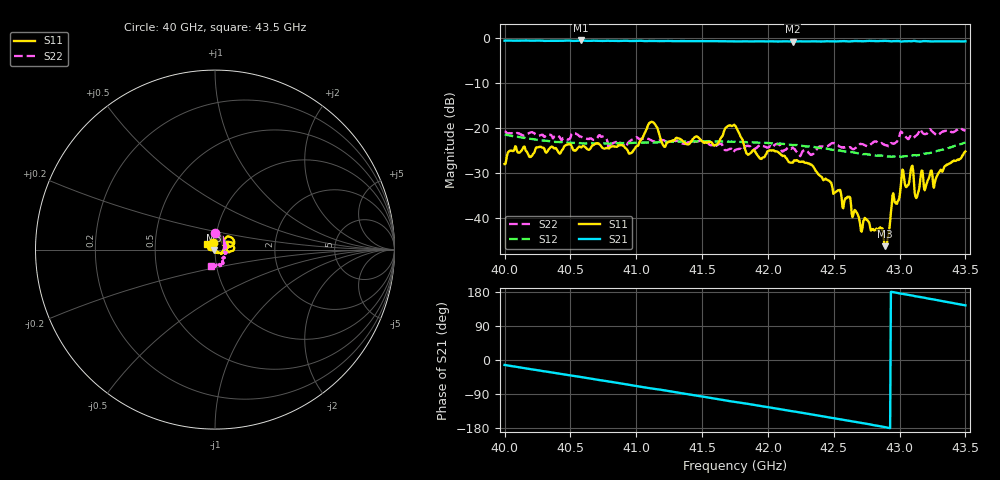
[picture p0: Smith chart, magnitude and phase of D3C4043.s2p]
! 4/15/2021 3:54:08 PM
! C:\USERS\DITOM\DESKTOP\SINGLE JUNCTION ISOLATOR DATA\40.0 - 43.5 GHZ (D3I4043).S2P
! CHANNEL.1
! TR.MEASUREMENT
! CORRECTED.DATA
# GHZ S RI R 50.0
! FREQ.GHZ  S11RE  S11IM  S21RE  S21IM  S12RE  S12IM  S22RE  S22IM
!; PortSelection: Port_12
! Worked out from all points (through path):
!   601 points, 40 GHz to 43.5 GHz, reference 50 ohm
!   highest |S21| = -0.51 dB at 40.58 GHz (marker M1); lowest = -0.8 dB at 42.19 GHz (marker M2)
!   lowest |S11| = -46.3 dB at 42.89 GHz (marker M3), VSWR 1.01, Z = 49.6 - j0.29 ohm
!   |S11| at or under -10 dB: start of sweep to end of sweep
!   |S22| runs from -26.3 to -20.0 dB; largest |S21 - S12| = 0.99
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40  -0.00855 0.0388  0.9137 -0.2125  0.00969 0.0841  0.000817 0.0918
40.07  -0.0225 0.0514  0.8949 -0.2746  0.0242 0.0771  0.00381 0.087
40.5775  0.0303 0.0531  0.6685 -0.6654  0.0679 -0.000592  0.0198 0.0778
40.58917  0.0262 0.0562  0.6595 -0.6727  0.0674 -0.00234  0.0214 0.076
40.95667  0.0437 0.0287  0.3771 -0.8511  0.0491 -0.0473  0.0415 0.0593
41.10833  0.1064 0.0453  0.245 -0.8987  0.0342 -0.0601  0.0403 0.0617
41.16667  0.0637 0.0687  0.2009 -0.9078  0.029 -0.0633  0.0446 0.0562
41.21333  0.0498 0.0368  0.1589 -0.9153  0.0235 -0.066  0.0443 0.0573
41.59833  0.0647 0.00393  -0.1918 -0.9055  -0.0238 -0.067  0.05 0.0371
41.75  0.1003 0.0361  -0.3215 -0.8626  -0.041 -0.0573  0.049 0.0288
41.84917  0.0496 0.00949  -0.4015 -0.8293  -0.0498 -0.0487  0.0571 0.0276
42.1875  0.037 -0.0177  -0.6505 -0.6462  -0.0643 -0.00714  0.0588 0.0151
42.33917  0.0321 -0.0202  -0.746 -0.5426  -0.0602 0.0142  0.0505 -0.00769
42.8875  -0.00386 -0.00292  -0.9311 -0.0456  0.00677 0.0483  0.045 -0.0464
42.91667  -0.00636 -0.0017  -0.93 -0.0134  0.0108 0.0469  0.0409 -0.0473
42.94583  -0.0173 -0.0029  -0.9238 0.00753  0.0151 0.0456  0.0392 -0.0547
43.0275  -0.0309 0.013  -0.9188 0.0901  0.0274 0.0398  0.0426 -0.0748
43.09167  -0.0364 0.00748  -0.912 0.1527  0.0359 0.0338  0.0245 -0.0738
43.1325  -0.0141 0.00984  -0.9013 0.1998  0.0408 0.0286  0.0259 -0.0801
43.16167  -0.0241 0.0183  -0.8909 0.2212  0.0436 0.025  0.0273 -0.0918
43.2725  -0.0234 0.0125  -0.8606 0.3326  0.0542 0.00807  0.0143 -0.084
43.5  -0.0452 0.0313  -0.7483 0.5391  0.0586 -0.036  -0.0209 -0.0914
